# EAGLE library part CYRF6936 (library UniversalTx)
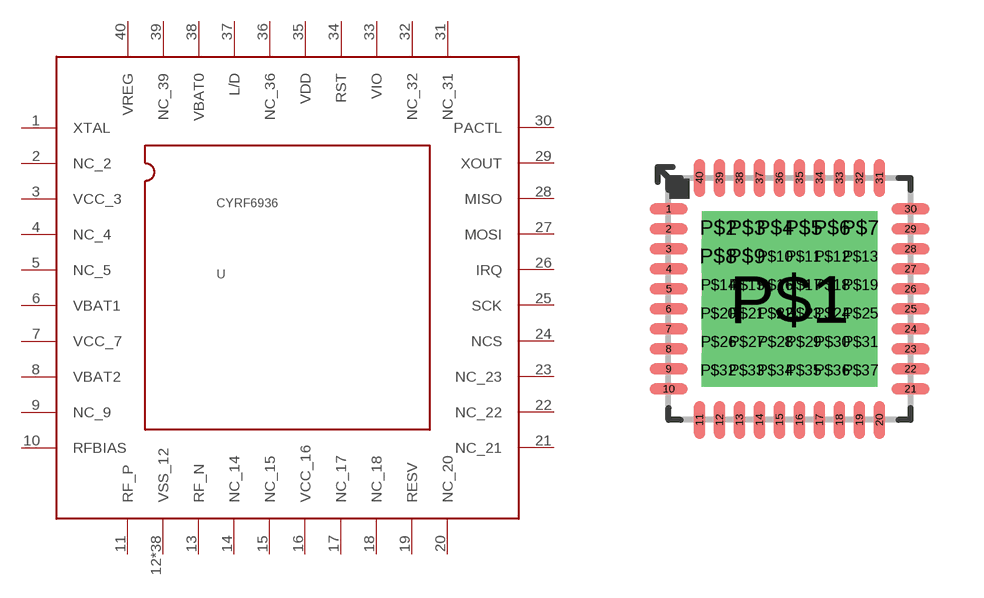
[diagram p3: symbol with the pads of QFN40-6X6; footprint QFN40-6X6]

Designator prefix -

## CYRF6936  [QFN40-6X6]
1  XTAL
2  NC_2
3  VCC_3
4  NC_4
5  NC_5
6  VBAT1
7  VCC_7
8  VBAT2
9  NC_9
10  RFBIAS
11  RF_P
12  VSS_12
13  RF_N
14  NC_14
15  NC_15
16  VCC_16
17  NC_17
18  NC_18
19  RESV
20  NC_20
21  NC_21
22  NC_22
23  NC_23
24  NCS
25  SCK
26  IRQ
27  MOSI
28  MISO
29  XOUT
30  PACTL
31  NC_31
32  NC_32
33  VIO
34  RST
35  VDD
36  NC_36
37  L/D
38  VBAT0
39  NC_39
40  VREG
P$1  VSS_12
P$2  VSS_12
P$3  VSS_12
P$4  VSS_12
P$5  VSS_12
P$6  VSS_12
P$7  VSS_12
P$8  VSS_12
P$9  VSS_12
P$10  VSS_12
P$11  VSS_12
P$12  VSS_12
P$13  VSS_12
P$14  VSS_12
P$15  VSS_12
P$16  VSS_12
P$17  VSS_12
P$18  VSS_12
P$19  VSS_12
P$20  VSS_12
P$21  VSS_12
P$22  VSS_12
P$23  VSS_12
P$24  VSS_12
P$25  VSS_12
P$26  VSS_12
P$27  VSS_12
P$28  VSS_12
P$29  VSS_12
P$30  VSS_12
P$31  VSS_12
P$32  VSS_12
P$33  VSS_12
P$34  VSS_12
P$35  VSS_12
P$36  VSS_12
P$37  VSS_12

## Footprint QFN40-6X6 (pad centres in mm)
RHA (S-PQFP-N40) 6 x 6 mm Source: http://focus.ti.com/lit/ds/symlink/tps65020.pdf
smd 0.95 x 0.28: 1 -3.025,2.25; 2 -3.025,1.75; 3 -3.025,1.25; 4 -3.025,0.75; 5 -3.025,0.25; 6 -3.025,-0.25; 7 -3.025,-0.75; 8 -3.025,-1.25; 9 -3.025,-1.75; 10 -3.025,-2.25; 21 3.025,-2.25; 22 3.025,-1.75; 23 3.025,-1.25; 24 3.025,-0.75; 25 3.025,-0.25; 26 3.025,0.25; 27 3.025,0.75; 28 3.025,1.25; 29 3.025,1.75; 30 3.025,2.25
smd 0.28 x 0.95: 11 -2.25,-3.025; 12 -1.75,-3.025; 13 -1.25,-3.025; 14 -0.75,-3.025; 15 -0.25,-3.025; 16 0.25,-3.025; 17 0.75,-3.025; 18 1.25,-3.025; 19 1.75,-3.025; 20 2.25,-3.025; 31 2.25,3.025; 32 1.75,3.025; 33 1.25,3.025; 34 0.75,3.025; 35 0.25,3.025; 36 -0.25,3.025; 37 -0.75,3.025; 38 -1.25,3.025; 39 -1.75,3.025; 40 -2.25,3.025
smd 4.2 x 4.2: P$1 0,0
drill 0.33 pad 0.686 square: P$2 -1.778,1.778; P$3 -1.067,1.778; P$4 -0.356,1.778; P$5 0.356,1.778; P$6 1.067,1.778; P$7 1.778,1.778; P$8 -1.783,1.067; P$9 -1.072,1.067; P$10 -0.361,1.067; P$11 0.351,1.067; P$12 1.062,1.067; P$13 1.773,1.067; P$14 -1.778,0.356; P$15 -1.067,0.356; P$16 -0.356,0.356; P$17 0.356,0.356; P$18 1.067,0.356; P$19 1.778,0.356; P$20 -1.783,-0.356; P$21 -1.072,-0.356; P$22 -0.361,-0.356; P$23 0.351,-0.356; P$24 1.062,-0.356; P$25 1.773,-0.356; P$26 -1.778,-1.067; P$27 -1.067,-1.067; P$28 -0.356,-1.067; P$29 0.356,-1.067; P$30 1.067,-1.067; P$31 1.778,-1.067; P$32 -1.783,-1.778; P$33 -1.072,-1.778; P$34 -0.361,-1.778; P$35 0.351,-1.778; P$36 1.062,-1.778; P$37 1.773,-1.778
